| IBIS file stm32l552_562_ufqfpn48.ibs
[IBIS ver]   4.2
[File name]  stm32l552_562_ufqfpn48.ibs
[File Rev]   1.0
[Date]   04-10-2019
[Source]   Data Created at STMicroelectronics
[Notes]   File originated from ELDO simulations.
[Disclaimer] This information is for modeling purpose only and is
   not guaranted.
   The information is subject to change without notice.
[Copyright]  Copyright 2019 STMicroelectronics Inc.
|   Component stm32l552_562_ufqfpn48
[Component] stm32l552_562_ufqfpn48
[Manufacturer] STMicroelectronics
[Package]
| variable   typ   min   max
R_pkg  0  NA  NA
L_pkg  0  NA  NA
C_pkg  0  NA  NA
[Pin]   signal_name   model_name R_pin L_pin C_pin
1 VBAT POWER
2 PC13 io8prog2m25m50m120m_sudq_ft
3 PC14-OSC32_IN io8prog2m25m50m120m_sudq_ft
4 PC15-OSC32_OUT io8prog2m25m50m120m_sudq_ft
5 PH0-OSC_IN io8prog2m25m50m120m_sudq_ft
6 PH1-OSC_OUT io8prog2m25m50m120m_sudq_ft
7 NRST ioreset_ft_v33
8 VSSA_VREF- GND
9 VDDA_VREF+ POWER
10 PA0 io8prog2m25m50m120m_sudq_ft
11 PA1 io8prog2m25m50m120m_sudq_ft
12 PA2 io8prog2m25m50m120m_sudq_ft
13 PA3 io8prog2m25m50m120m_sudq_ft
14 PA4 io8prog2m25m50m120m_sudq_ft
15 PA5 io8prog2m25m50m120m_sudq_ft
16 PA6 io8prog2m25m50m120m_sudq_ft
17 PA7 io8prog2m25m50m120m_sudq_i2c_ft
18 PB0 io8prog2m25m50m120m_sudq_ft
19 PB1 io8prog2m25m50m120m_sudq_ft
20 PB2 io8prog2m25m50m120m_sudq_ft
21 PB10 io8prog2m25m50m120m_sudq_i2c_ft
22 PB11 io8prog2m25m50m120m_sudq_i2c_ft
23 VSS GND
24 VDD POWER
25 PB12 io8prog2m25m50m120m_sudq_ft
26 PB13 io8prog2m25m50m120m_sudq_i2c_ft
27 PB14 io8prog2m25m50m120m_sudq_i2c_ft
28 PB15 io6usb_bmc_pd_cc_ft
29 PA8 io8prog2m25m50m120m_sudq_i2c_ft
30 PA9 io8prog2m25m50m120m_sudq_ft
31 PA10 io8prog2m25m50m120m_sudq_ft
32 PA11 io8usblsfs_otg2
33 PA12 io8usblsfs_otg2
34 PA13 io8prog2m25m50m120m_sudq_ft
35 VSS GND
36 VDD POWER
37 PA14 io8prog2m25m50m120m_sudq_i2c_ft
38 PA15 io6usb_bmc_pd_cc_ft
39 PB3 io8prog2m25m50m120m_sudq_ft
40 PB4 io8prog2m25m50m120m_sudq_i2c_ft
41 PB5 io8prog2m25m50m120m_sudq_ft
42 PB6 io8prog2m25m50m120m_sudq_i2c_ft
43 PB7 io8prog2m25m50m120m_sudq_i2c_ft
44 PH3-BOOT0 io8prog2m25m50m120m_sudq_ft
45 PB8 io8prog2m25m50m120m_sudq_i2c_ft
46 PB9 io8prog2m25m50m120m_sudq_i2c_ft
47 VSS GND
48 VDD POWER
[Model Selector] io6usb_bmc_pd_cc_ft
usb_bmc_emit_pdccpd  "BMC PD emitter  + PD"
usb_bmc_emit_pdcc3a0  "BMC PD emitter  + 3rd PU"
usb_bmc_emit_pdcc1a5  "BMC PD emitter  + 2nd PU"
usb_bmc_emit_pdccusb  "BMC PD emitter  + 1st PU"
usb_bmc_emit  "BMC PD emitter "
io2_pdcc_ft_3v3_lowspeed  "GPIO-3.3V range - low speed"
io2_pdcc_ft_3v3_mediumspeed  "GPIO-3.3V range - medium speed"
io2_pdcc_ft_3v3_lowspeed_pu  "GPIO-3.3V range - low speed - pull up"
io2_pdcc_ft_3v3_mediumspeed_pu  "GPIO-3.3V range - medium speed - pull up"
io2_pdcc_ft_3v3_lowspeed_pd  "GPIO-3.3V range - low speed - pull down"
io2_pdcc_ft_3v3_mediumspeed_pd  "GPIO-3.3V range - medium speed - pull down"
io2_pdcc_ft_1v8_lowspeed  "GPIO-1.8V range - low speed"
io2_pdcc_ft_1v8_mediumspeed  "GPIO-1.8V range - medium speed"
io2_pdcc_ft_1v8_lowspeed_pu  "GPIO-1.8V range - low speed - pull up"
io2_pdcc_ft_1v8_mediumspeed_pu  "GPIO-1.8V range - medium speed - pull up"
io2_pdcc_ft_1v8_lowspeed_pd  "GPIO-1.8V range - low speed - pull down"
io2_pdcc_ft_1v8_mediumspeed_pd  "GPIO-1.8V range - medium speed - pull down"
io2_pdcc_ft_1v2_lowspeed  "GPIO-1.2V range - low speed"
io2_pdcc_ft_1v2_mediumspeed  "GPIO-1.2V range - medium speed"
io2_pdcc_ft_1v2_lowspeed_pu  "GPIO-1.2V range - low speed - pull up"
io2_pdcc_ft_1v2_mediumspeed_pu  "GPIO-1.2V range - medium speed - pull up"
io2_pdcc_ft_1v2_lowspeed_pd  "GPIO-1.2V range - low speed - pull down"
io2_pdcc_ft_1v2_mediumspeed_pd  "GPIO-1.2V range - medium speed - pull down"
[Model Selector] io8prog2m25m50m120m_sudq_ft
iols8p_sudq_ft_pd_lv  "IO low speed, PD=40kOhm - 1P8V"
iols8p_sudq_ft_pu_lv  "IO low speed, PU=40kOhm - 1P8V"
iols8p_sudq_ft_lv  "IO low speed - 1P8V"
iols8p_sudq_ft_pd  "IO low speed, PD=40kOhm - 3P3V"
iols8p_sudq_ft_pu  "IO low speed, PU=40kOhm - 3P3V"
iols8p_sudq_ft  "IO low speed - 3P3V"
iofs8p_sudq_ft_pd_lv  "IO full speed, PD=40kOhm - 1P8V"
iofs8p_sudq_ft_pu_lv  "IO full speed, PU=40kOhm - 1P8V"
iofs8p_sudq_ft_lv  "IO full speed - 1P8V"
iofs8p_sudq_ft_pd  "IO full speed, PD=40kOhm - 3P3V"
iofs8p_sudq_ft_pu  "IO full speed, PU=40kOhm - 3P3V"
iofs8p_sudq_ft  "IO full speed - 3P3V"
ioms8p_sudq_ft_pd_lv  "IO medium speed, PD=40kOhm - 1P8V"
ioms8p_sudq_ft_pu_lv  "IO medium speed, PU=40kOhm - 1P8V"
ioms8p_sudq_ft_lv  "IO medium speed - 1P8V"
ioms8p_sudq_ft_pd  "IO medium speed, PD=40kOhm - 3P3V"
ioms8p_sudq_ft_pu  "IO medium speed, PU=40kOhm - 3P3V"
ioms8p_sudq_ft  "IO medium speed - 3P3V"
iohs8p_sudq_ft_pd_lv  "IO high speed, PD=40kOhm - 1P8V"
iohs8p_sudq_ft_pu_lv  "IO high speed, PU=40kOhm - 1P8V"
iohs8p_sudq_ft_lv  "IO high speed - 1P8V"
iohs8p_sudq_ft_pd  "IO high speed, PD=40kOhm - 3P3V"
iohs8p_sudq_ft_pu  "IO high speed, PU=40kOhm - 3P3V"
iohs8p_sudq_ft  "IO high speed - 3P3V"
[Model Selector] io8prog2m25m50m120m_sudq_i2c_ft
io8prog_1v8_i2c_pd  "5V Tol GPIO 1.8V range i2c functionality with pull down"
io8prog_1v8_i2c_pu  "5V Tol GPIO 1.8V range i2c functionality with pull up"
io8prog_1v8_i2c  "5V Tol GPIO 1.8V range i2c functionality"
io8prog_3v3_i2c_pd  "5V Tol GPIO 3.3V range i2c functionality with pull down"
io8prog_3v3_i2c_pu  "5V Tol GPIO 3.3V range i2c functionality with pull up"
io8prog_3v3_i2c  "5V Tol GPIO 3.3V range i2c functionality"
iols8p_sudq_ft_pd_lv  "IO low speed, PD=40kOhm - 1P8V"
iols8p_sudq_ft_pu_lv  "IO low speed, PU=40kOhm - 1P8V"
iols8p_sudq_ft_lv  "IO low speed - 1P8V"
iols8p_sudq_ft_pd  "IO low speed, PD=40kOhm - 3P3V"
iols8p_sudq_ft_pu  "IO low speed, PU=40kOhm - 3P3V"
iols8p_sudq_ft  "IO low speed - 3P3V"
iofs8p_sudq_ft_pd_lv  "IO full speed, PD=40kOhm - 1P8V"
iofs8p_sudq_ft_pu_lv  "IO full speed, PU=40kOhm - 1P8V"
iofs8p_sudq_ft_lv  "IO full speed - 1P8V"
iofs8p_sudq_ft_pd  "IO full speed, PD=40kOhm - 3P3V"
iofs8p_sudq_ft_pu  "IO full speed, PU=40kOhm - 3P3V"
iofs8p_sudq_ft  "IO full speed - 3P3V"
ioms8p_sudq_ft_pd_lv  "IO medium speed, PD=40kOhm - 1P8V"
ioms8p_sudq_ft_pu_lv  "IO medium speed, PU=40kOhm - 1P8V"
ioms8p_sudq_ft_lv  "IO medium speed - 1P8V"
ioms8p_sudq_ft_pd  "IO medium speed, PD=40kOhm - 3P3V"
ioms8p_sudq_ft_pu  "IO medium speed, PU=40kOhm - 3P3V"
ioms8p_sudq_ft  "IO medium speed - 3P3V"
iohs8p_sudq_ft_pd_lv  "IO high speed, PD=40kOhm - 1P8V"
iohs8p_sudq_ft_pu_lv  "IO high speed, PU=40kOhm - 1P8V"
iohs8p_sudq_ft_lv  "IO high speed - 1P8V"
iohs8p_sudq_ft_pd  "IO high speed, PD=40kOhm - 3P3V"
iohs8p_sudq_ft_pu  "IO high speed, PU=40kOhm - 3P3V"
iohs8p_sudq_ft  "IO high speed - 3P3V"
[Model Selector] io8usblsfs_otg2
usb_ls_pd  "USB Low Speed mode - Pull Down"
usb_ls_pu2  "USB Low Speed mode - Pull up 2"
usb_ls_pu  "USB Low Speed mode - Pull up"
usb_fs  "USB Low Speed mode"
usb_fs_pd  "USB Full Speed mode - Pull Down"
usb_fs_pu2  "USB Full Speed mode - Pull up 2"
usb_fs_pu  "USB Full Speed mode - Pull up"
[Model Selector] ioreset_ft_v33
ioreset_1v2_pu  "RESET 1.2V range with PU"
ioreset_1v2  "RESET 1.2V range"
ioreset_1v8_pu  "RESET 1.8V range with PU"
ioreset_1v8  "RESET 1.8V range"
ioreset_3v3_pu  "RESET 3.3V range with PU"
ioreset_3v3  "RESET 3.3V range"
| Models and submodels in the file (66): usb_bmc_emit_pdccpd (I/O), usb_bmc_emit_pdcc3a0 (I/O), usb_bmc_emit_pdcc1a5 (I/O), usb_bmc_emit_pdccusb (I/O), usb_bmc_emit (I/O), io2_pdcc_ft_3v3_lowspeed (I/O), io2_pdcc_ft_3v3_mediumspeed (I/O), io2_pdcc_ft_3v3_lowspeed_pu (I/O), io2_pdcc_ft_3v3_mediumspeed_pu (I/O), io2_pdcc_ft_3v3_lowspeed_pd (I/O), io2_pdcc_ft_3v3_mediumspeed_pd (I/O), io2_pdcc_ft_1v8_lowspeed (I/O), io2_pdcc_ft_1v8_mediumspeed (I/O), io2_pdcc_ft_1v8_lowspeed_pu (I/O), io2_pdcc_ft_1v8_mediumspeed_pu (I/O), io2_pdcc_ft_1v8_lowspeed_pd (I/O), io2_pdcc_ft_1v8_mediumspeed_pd (I/O), io2_pdcc_ft_1v2_lowspeed (I/O), io2_pdcc_ft_1v2_mediumspeed (I/O), io2_pdcc_ft_1v2_lowspeed_pu (I/O), io2_pdcc_ft_1v2_mediumspeed_pu (I/O), io2_pdcc_ft_1v2_lowspeed_pd (I/O), io2_pdcc_ft_1v2_mediumspeed_pd (I/O), iols8p_sudq_ft_pd_lv (I/O), iols8p_sudq_ft_pu_lv (I/O), iols8p_sudq_ft_lv (I/O), iols8p_sudq_ft_pd (I/O), iols8p_sudq_ft_pu (I/O), iols8p_sudq_ft (I/O), iofs8p_sudq_ft_pd_lv (I/O), iofs8p_sudq_ft_pu_lv (I/O), iofs8p_sudq_ft_lv (I/O), iofs8p_sudq_ft_pd (I/O), iofs8p_sudq_ft_pu (I/O), iofs8p_sudq_ft (I/O), ioms8p_sudq_ft_pd_lv (I/O), ioms8p_sudq_ft_pu_lv (I/O), ioms8p_sudq_ft_lv (I/O), ioms8p_sudq_ft_pd (I/O), ioms8p_sudq_ft_pu (I/O), ioms8p_sudq_ft (I/O), iohs8p_sudq_ft_pd_lv (I/O), iohs8p_sudq_ft_pu_lv (I/O), iohs8p_sudq_ft_lv (I/O), iohs8p_sudq_ft_pd (I/O), iohs8p_sudq_ft_pu (I/O), iohs8p_sudq_ft (I/O), io8prog_1v8_i2c_pd (I/O_open_drain), io8prog_1v8_i2c_pu (I/O_open_drain), io8prog_1v8_i2c (I/O_open_drain), io8prog_3v3_i2c_pd (I/O_open_drain), io8prog_3v3_i2c_pu (I/O_open_drain), io8prog_3v3_i2c (I/O_open_drain), usb_ls_pd (I/O), usb_ls_pu2 (I/O), usb_ls_pu (I/O), usb_fs (I/O), usb_fs_pd (I/O), usb_fs_pu2 (I/O), usb_fs_pu (I/O), ioreset_1v2_pu (I/O_open_drain), ioreset_1v2 (I/O_open_drain), ioreset_1v8_pu (I/O_open_drain), ioreset_1v8 (I/O_open_drain), ioreset_3v3_pu (I/O_open_drain), ioreset_3v3 (I/O_open_drain)
